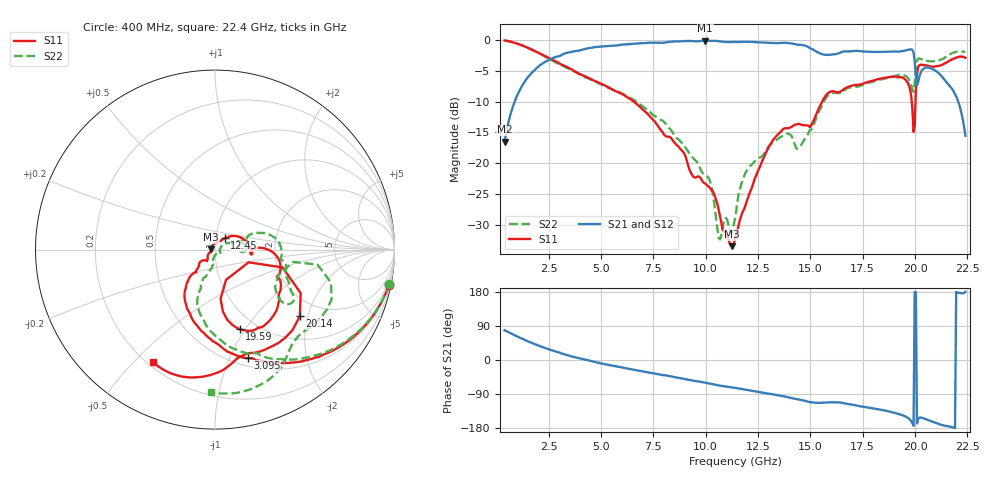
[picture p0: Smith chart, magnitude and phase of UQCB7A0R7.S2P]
!  Part Number  UQCB7A0R7	Mounting Orientation: Vertical
!  Description: RF capacitors
!  Application: Coupling, Bypass, Tuning, DC Block
!  Filters, Matching
# GHZ S DB R 50
! Freq  |S11|  S11 Ph  |S21|  S21 Ph  |S12|  S12 Ph  |S22|  S22 Ph
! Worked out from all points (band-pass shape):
!   401 points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, 400 MHz to 22.4 GHz, reference 50 ohm
!   highest |S21| = -0.13 dB at 9.97 GHz (marker M1); lowest = -16.5 dB at 400 MHz (marker M2)
!   |S21| within 3 dB of the highest: 2.588 GHz to 19.97 GHz (17.38 GHz wide, 154 % of centre)
!   lowest |S11| = -33.4 dB at 11.23 GHz (marker M3), VSWR 1.04, Z = 47.9 + j0.245 ohm
!   |S11| at or under -10 dB: 6.571 GHz to 15.56 GHz (8.991 GHz wide, 81.2 % of centre); 19.84 GHz to 20.02 GHz (180.2 MHz wide, 0.904 % of centre)
!   |S22| runs from -32.3 to -0.1 dB; largest |S21 - S12| = 0.0035
!   S11 on the Smith chart (normalised r, x): 400 MHz: 0.63, -9.87; 3.095 GHz: 0.58, -1.17; 12.45 GHz: 1.11, +0.14; 19.59 GHz: 0.83, -0.94; 20.14 GHz: 1.53, -1.79; 22.4 GHz: 0.22, -0.57
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0.4  -0.11 -11.5  -16.51 78.5  -16.52 78.5  -0.10 -11.1
1.39  -1.11 -38.0  -6.61 52.3  -6.62 52.3  -1.12 -36.9
3.095  -4.00 -73.2  -2.50 17.4  -2.51 17.4  -4.21 -69.3
4.085  -5.68 -89.4  -1.62 3.2  -1.63 3.2  -5.76 -85.3
7.77  -14.19 -132.9  -0.45 -38.2  -0.45 -38.2  -12.76 -110.3
9.97  -23.26 -126.6  -0.13 -60.0  -0.13 -59.9  -21.85 -92.4
10.63  -27.67 -148.0  -0.23 -67.1  -0.23 -67.2  -32.11 -69.9
11.235  -33.41 173.1  -0.35 -72.0  -0.36 -72.1  -31.35 -2.5
11.4  -32.28 136.8  -0.34 -73.5  -0.34 -73.5  -28.89 23.0
11.785  -27.72 71.8  -0.31 -77.0  -0.31 -77.1  -22.51 28.3
12.445  -21.63 49.2  -0.40 -83.6  -0.39 -83.7  -19.33 20.2
13.655  -14.61 12.9  -0.49 -94.8  -0.48 -94.8  -15.62 9.3
14.425  -13.61 -5.2  -0.79 -103.8  -0.79 -103.8  -17.54 7.0
15.085  -13.52 0.1  -1.50 -111.8  -1.50 -111.9  -14.33 21.2
15.91  -8.48 -14.2  -2.41 -111.7  -2.42 -111.7  -8.79 4.3
18.77  -6.03 -52.8  -1.91 -135.9  -1.91 -136.1  -6.08 -29.7
19.595  -6.66 -72.7  -1.68 -150.7  -1.67 -150.9  -5.98 -37.1
19.925  -14.92 -70.0  -2.11 -173.6  -2.10 -173.8  -8.41 -21.5
20.145  -4.42 -38.2  -6.82 -156.1  -6.81 -156.3  -3.03 -22.9
20.42  -4.10 -61.6  -4.64 -154.2  -4.62 -154.3  -3.26 -37.8
21.245  -4.09 -79.3  -5.80 -171.0  -5.79 -171.1  -3.19 -52.9
22.4  -2.91 -119.1  -15.54 179.9  -15.56 179.6  -1.98 -91.8
